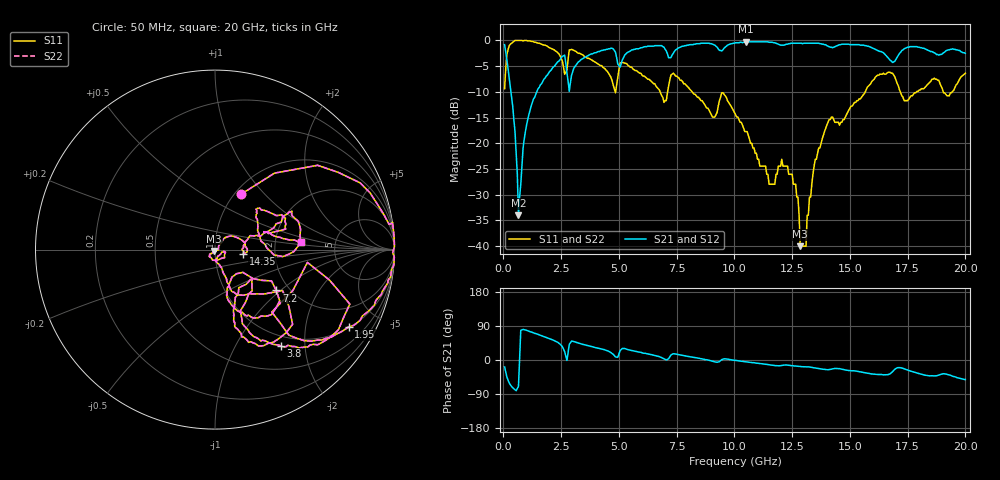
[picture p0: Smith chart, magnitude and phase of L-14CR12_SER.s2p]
#	mhz	s	ma	r	50
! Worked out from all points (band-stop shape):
!   400 points, 50 MHz to 20 GHz, reference 50 ohm
!   highest |S21| = -0.26 dB at 10.5 GHz (marker M1); lowest = -34.0 dB at 650 MHz (marker M2)
!   |S21| within 3 dB of the highest: 7.259 GHz to 16.63 GHz (9.374 GHz wide, 78.5 % of centre); 17.04 GHz to end of sweep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
!   lowest |S11| = -40.0 dB at 12.85 GHz (marker M3), VSWR 1.02, Z = 49.4 - j0.816 ohm
!   |S11| at or under -10 dB: 8.169 GHz to 15.67 GHz (7.497 GHz wide, 62.9 % of centre); 17.18 GHz to 17.88 GHz (697.2 MHz wide, 3.98 % of centre); 19.04 GHz to 19.43 GHz (392.1 MHz wide, 2.04 % of centre)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
!   |S22| runs from -40.0 to 0.0 dB; largest |S21 - S12| = 0
!   S11 on the Smith chart (normalised r, x): 50 MHz: 1.07, +0.74; 1.95 GHz: 1.04, -3.44; 3.8 GHz: 0.84, -1.56; 7.2 GHz: 1.71, -0.94; 14.35 GHz: 1.37, -0.07; 20 GHz: 2.81, +0.30
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50  0.34 64.9  0.91 -18.3  0.91 -18.3  0.34 64.9
250  0.89 24.7  0.43 -60.8  0.43 -60.8  0.89 24.7
500  1 8.5  0.13 -78.5  0.13 -78.5  1 8.5
650  1 5.1  0.02 -69.6  0.02 -69.6  1 5.1
1050  0.99 -6.4  0.17 77.4  0.17 77.4  0.99 -6.4
1950  0.86 -30.0  0.48 57.4  0.48 57.4  0.86 -30.0
2550  0.63 -49.2  0.7 35.4  0.7 35.4  0.63 -49.2
2750  0.52 -7.9  0.48 -1.2  0.48 -1.2  0.52 -7.9
3400  0.73 -48.3  0.66 41.8  0.66 41.8  0.73 -48.3
3800  0.65 -55.7  0.74 35.7  0.74 35.7  0.65 -55.7
6700  0.34 -71.8  0.89 9.6  0.89 9.6  0.34 -71.8
7200  0.41 -33.7  0.68 8.2  0.68 8.2  0.41 -33.7
10050  0.19 -69.7  0.95 -1.2  0.95 -1.2  0.19 -69.7
10500  0.13 -70.7  0.97 -5.0  0.97 -5.0  0.13 -70.7
11500  0.04 -68.8  0.96 -12.4  0.96 -12.4  0.04 -68.8
12500  0.05 -130.3  0.94 -15.0  0.94 -15.0  0.05 -130.3
12850  0.01 -124.4  0.94 -17.4  0.94 -17.4  0.01 -124.4
13100  0.01 -23.8  0.94 -18.1  0.94 -18.1  0.01 -23.8
13350  0.04 47.0  0.94 -19.8  0.94 -19.8  0.04 47.0
14350  0.16 -9.1  0.87 -22.2  0.87 -22.2  0.16 -9.1
16700  0.49 16.1  0.66 -37.4  0.66 -37.4  0.49 16.1
20000  0.48 4.9  0.75 -51.5  0.75 -51.5  0.48 4.9
